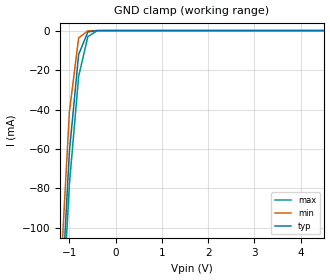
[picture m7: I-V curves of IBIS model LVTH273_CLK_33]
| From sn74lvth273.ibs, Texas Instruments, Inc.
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|   Model LVTH273_CLK_33
[Model]   LVTH273_CLK_33
Model_type  Input
Polarity   Non-Inverting
Vinl = 0.8V
Vinh = 2.0V
| variable   typ   min   max
C_comp   4pf   NA   NA
[Temperature Range]   40   -25   100
| Ambient temperature   25   -40   85
[Voltage range]   3.3   3.0   3.6
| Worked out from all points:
|   GND clamp passes 1 mA (typ) near -0.61 V on its own axis
[GND Clamp]
|   Voltage   I(typ)   I(min)   I(max)
-5V       -2.435A    -2.775A    -2.162A
-1.2V     -148.9mA   -127.9mA   -163.3mA
-1V       -61.21mA   -41.17mA   -77.93mA
-800mV    -12.04mA   -3.719mA   -23.11mA
-600mV    -698.8uA   -96.64uA   -3.029mA
-400mV    -3.355uA   -90.86nA   -94.19uA
5V        560.8pA    293.9nA    275.9pA
